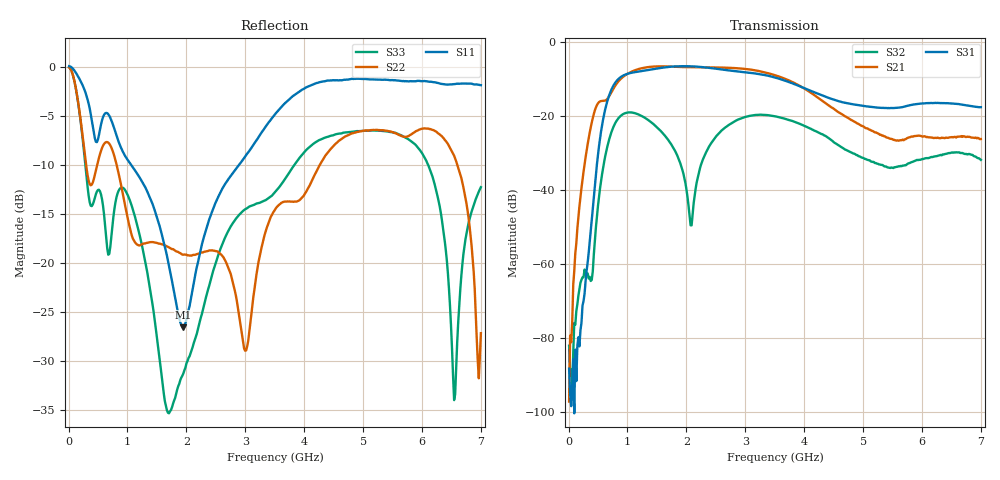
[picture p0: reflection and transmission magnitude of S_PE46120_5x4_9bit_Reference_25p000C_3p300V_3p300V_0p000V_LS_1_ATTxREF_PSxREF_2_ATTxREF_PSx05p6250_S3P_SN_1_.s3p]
! Device ID: PE46120_5x4_9bit_Reference
! Device ID: PE46120_5x4_9bit_Reference
! File Path: z:\PE46120_5x4_9bit_Reference\MPAC_Yi\new_12port\25p000C\3p300\LS_1_ATTxREF_PSxREF_2_ATTxREF_PSx05p6250\PE46120_5x4_9bit_Reference_25p000C_3p300V_3p300V_0p000V_LS_1_ATTxREF_PSxREF_2_ATTxREF_PSx05p6250_S3P_SN_1_.s3p
! Serial: 1
! Lot:
! Temp: 25.000C
! VDD: 3.300
! VSS: 0.000
! Control_Hi: 3.300
! Control_Lo: 0.000
! Logic State: LS_1_ATTxREF_PSxREF_2_ATTxREF_PSx05p6250
! Port 1: RFin
! Port 2: RFout1
! Port 3: RFout2
! ThroughPath:1-3
! IDD: -0.0005477357
! ISS: 0
! Comment:
#  Hz  S  RI  R  50
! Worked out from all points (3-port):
!   401 points, 10 MHz to 7 GHz, reference 50 ohm
!   strongest paths, dB at 10 MHz, 1.758 GHz, 3.505 GHz, 5.253 GHz, 7 GHz:
!     S31: -88.3, -6.7, -9.6, -17.7, -17.6
!     S21: -97.2, -6.7, -9.0, -24.7, -26.2
!     S32: -82.1, -28.0, -20.1, -32.9, -31.9
!   lowest |S11| = -26.5 dB at 1.95 GHz (marker M1), VSWR 1.10, Z = 54.8 + j1.1 ohm
!   |S11| at or under -10 dB: 1.065 GHz to 2.892 GHz (1.828 GHz wide, 92.4 % of centre)
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1e7  1.001 -0.1151  0.000121 5.18e-05  -0.000115 1.06e-05
     1.34e-05 -3.23e-06  0.9875 -0.0964  5.78e-06 7.76e-05
     -9.24e-06 -3.73e-05  -7.65e-05 -1.75e-05  0.9875 -0.0965
2.37175e8  -0.4709 -0.6568  -0.0127 -0.00475  9.5e-05 0.000184
           -0.0128 -0.00485  -0.2837 -0.3499  -0.000289 0.00059
           0.000107 0.000251  -0.00024 0.000613  -0.2749 -0.3406
4.6435e8  -0.4082 -0.0749  -0.0548 0.1161  0.016 0.00144
          -0.0554 0.1178  0.1377 0.2625  -0.00204 0.00219
          0.0161 0.00144  -0.00207 0.00229  0.1795 0.1346
9.187e8  -0.2853 0.2376  0.3287 -0.0245  -0.1156 0.3238
         0.3329 -0.025  -0.0335 -0.2255  -0.065 0.0811
         -0.1167 0.328  -0.0657 0.0821  0.0751 -0.2304
1.949725e9  0.046 0.0101  -0.3895 0.2302  -0.2807 -0.3709
            -0.3936 0.2336  -0.0967 0.053  0.000315 0.0164
            -0.2846 -0.3751  0.000435 0.0167  -0.00228 -0.0273
2.806e9  -0.096 -0.2755  0.4285 0.0947  -0.0589 0.3958
         0.4339 0.095  0.0709 -0.0278  0.0205 0.08
         -0.0588 0.4008  0.0207 0.0808  0.0764 0.1432
3.505e9  -0.4183 -0.3918  -0.0922 -0.3383  0.3267 -0.00163
         -0.094 -0.3428  0.0612 0.1768  -0.0051 -0.0975
         0.3307 -0.00225  -0.00553 -0.0989  0.0579 -0.2223
5.899075e9  -0.5247 0.6617  0.0527 -0.00524  -0.0894 0.1113
            0.0535 -0.00546  0.4402 0.1656  -0.00517 -0.0246
            -0.0897 0.1127  -0.00534 -0.0245  0.3815 -0.1137
6.54565e9  -0.271 0.7705  0.0187 -0.0474  0.075 0.1241
           0.0182 -0.0487  0.272 -0.2244  -0.0157 0.0273
           0.0768 0.1256  -0.0165 0.0277  0.0199 -0.00204
7e9  -0.1009 0.8002  -0.0279 -0.0389  0.1236 0.038
     -0.0285 -0.0395  -0.0336 0.0284  0.0251 0.00595
     0.1259 0.0378  0.0249 0.00534  0.0869 0.2276
